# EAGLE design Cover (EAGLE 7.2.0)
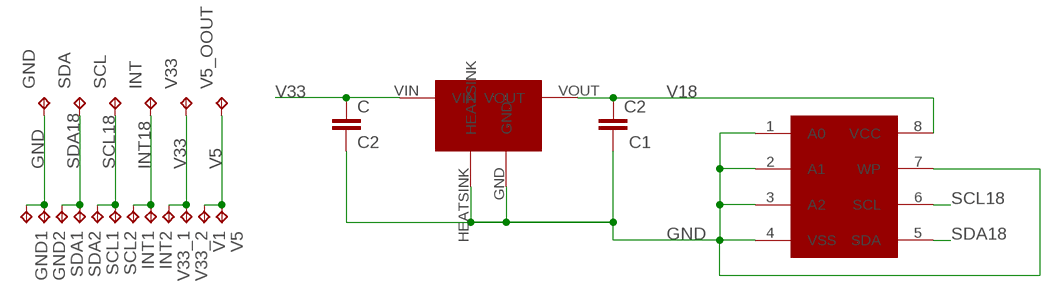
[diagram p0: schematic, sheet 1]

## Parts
C  C2  C-EUC0603  [C0603]
C2  C1  C-EUC0603  [C0603]
GND  TPTP20SQ  [TP20SQ]
GND1  TPTP20SQ  [TP20SQ]
GND2  TPTP20SQ  [TP20SQ]
INT  TPTP20SQ  [TP20SQ]
INT1  TPTP20SQ  [TP20SQ]
INT2  TPTP20SQ  [TP20SQ]
SCL  TPTP20SQ  [TP20SQ]
SCL1  TPTP20SQ  [TP20SQ]
SCL2  TPTP20SQ  [TP20SQ]
SDA  TPTP20SQ  [TP20SQ]
SDA1  SDA  TPTP20SQ  [TP20SQ]
SDA2  SDA  TPTP20SQ  [TP20SQ]
U$1  CAT24  [CAT24]
U$2  MCP1700-DFN6  [DFN6-2X2]
V1  V5  TPTP20SQ  [TP20SQ]
V5  V5  TPTP20SQ  [TP20SQ]
V5_OOUT  TPTP20SQ  [TP20SQ]
V33  TPTP20SQ  [TP20SQ]
V33_1  TPTP20SQ  [TP20SQ]
V33_2  TPTP20SQ  [TP20SQ]

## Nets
GND: C2.2 C.2 GND1.TP GND2.TP GND.TP U$1.1(A0) U$1.2(A1) U$1.3(A2) U$1.4(VSS) U$1.7(WP) U$2.GND U$2.HEATSINK
INT18: INT1.TP INT2.TP INT.TP
SCL18: SCL1.TP SCL2.TP SCL.TP U$1.6(SCL)
SDA18: SDA1.TP SDA2.TP SDA.TP U$1.5(SDA)
V5: V1.TP V5.TP V5_OOUT.TP
V18: C2.1 U$1.8(VCC) U$2.VOUT
V33: C.1 U$2.VIN V33.TP V33_1.TP V33_2.TP

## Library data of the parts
C C2 = rcl:C-EU: CAPACITOR, European symbol
GND GND1 GND2 INT INT1 INT2 SCL SCL1 SCL2 SDA SDA1 SDA2 V1 V5 V5_OOUT V33 V33_1 V33_2 = testpad:TP: Test pad
U$1 = cat24:CAT24
U$2 = MCP1700_DFN6-2x2:MCP1700-DFN6

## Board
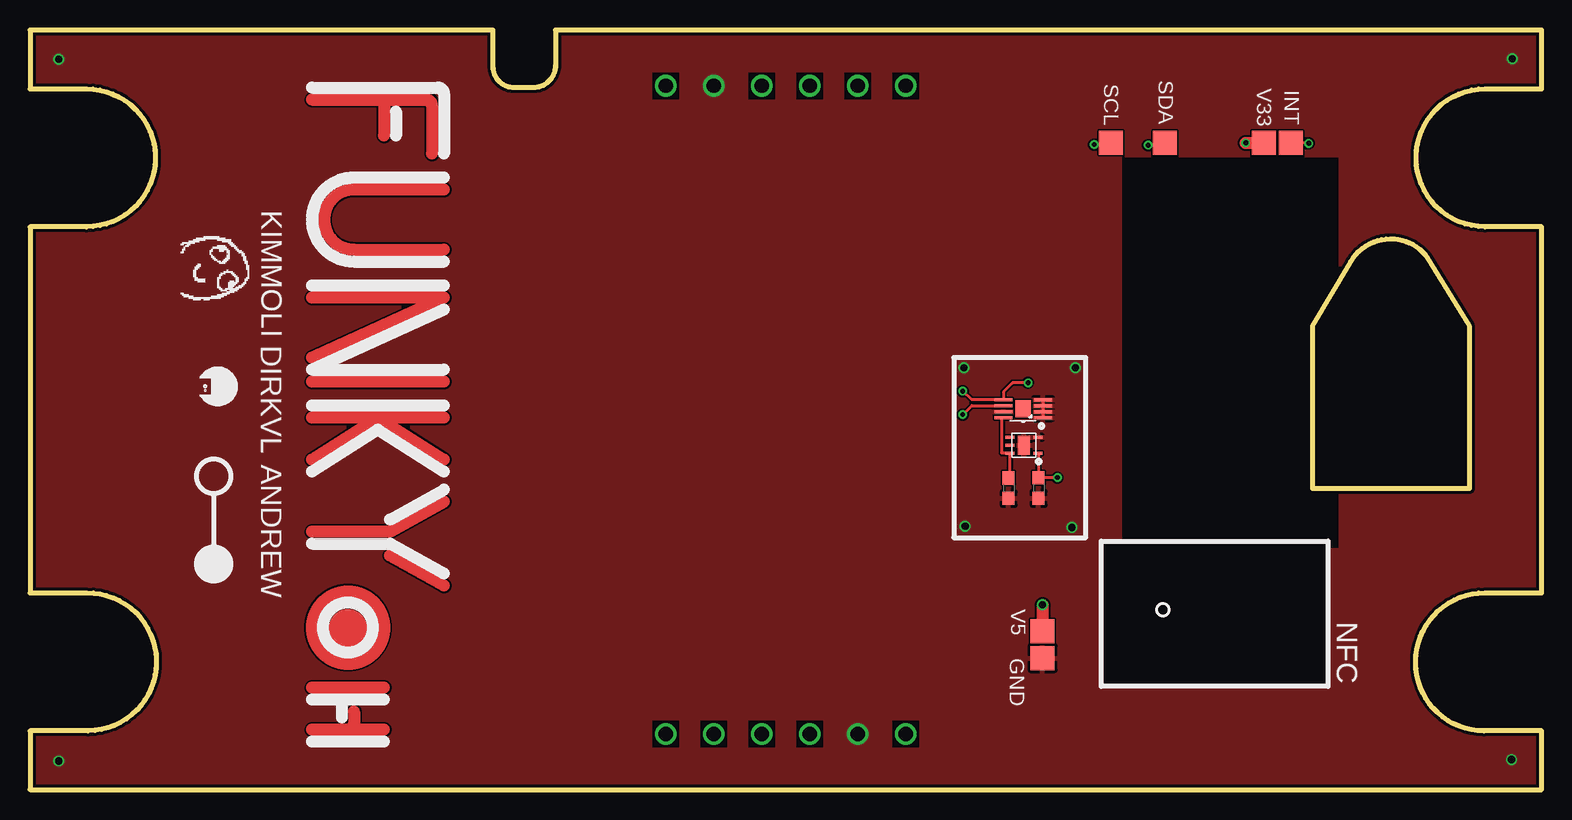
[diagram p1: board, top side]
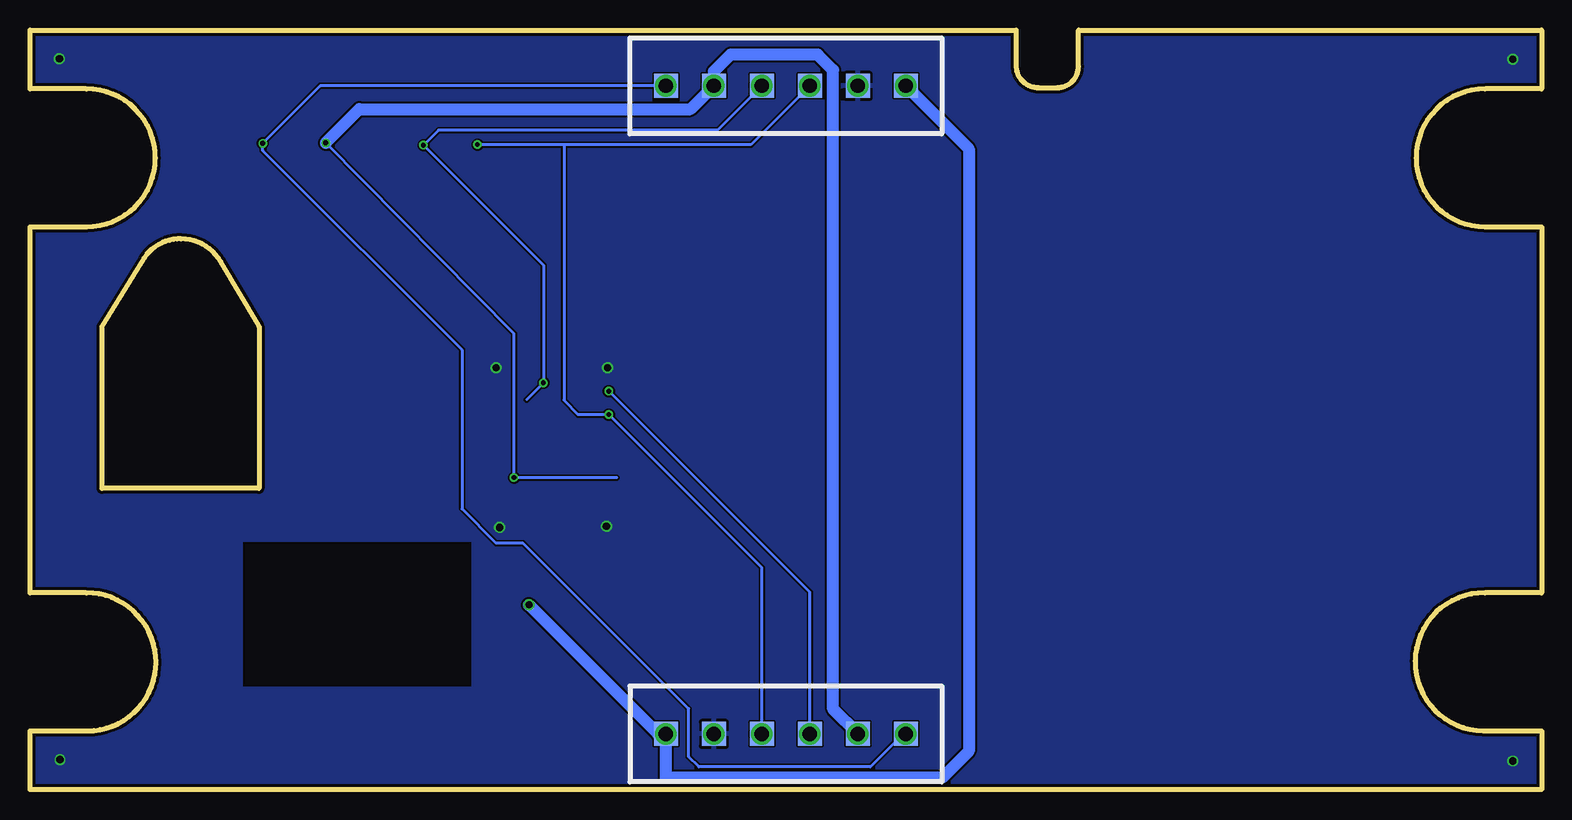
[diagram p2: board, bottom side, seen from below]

Size 126 x 63.3 mm. Coordinates in mm from the lower left corner, seen from the top.
Outline: 0,0 126,0 126,4.9 121.2,4.9 arc-90 115.5,10.6 arc-90 121.3,16.4 126,16.4 126,46.9 121.3,46.9 arc-180 121.3,58.4 126,58.4 126,63.3 43.8,63.3 43.8,60.35 arc-90 41.95,58.5 40.35,58.5 arc-90 38.6,60.25 38.6,63.3 0,63.3 0,58.4 4.7,58.4 arc-180 4.7,46.9 0,46.9 0,16.4 4.72,16.4 arc-180 4.85,4.9 0,4.9 0,0
Outline: 106.9,38.6 106.9,25.1 120,25.1 120,38.6 116.5,44.3 arc56 113.4,45.9 arc59 110.1,44 106.9,38.6
Copper layers (1*16): Top 0.035mm / dielectric 1.5mm / Bottom 0.035mm
Design rules "ITEADstudio_DRC": minimum track width 6mil, minimum drill 12mil, track to track 6mil, track to pad 6mil, pad to pad 6mil, via to via 6mil, smd to smd 0mil, copper to edge 10mil, drill to drill 10mil, minimum pad ring 10mil, minimum via ring 6mil, stop-mask expansion 2mil, vias tented up to drill 100mil, thermal gap 10mil
tRestrict: area 51.9,3.6 to 54.1,5.8; area 55.9,3.6 to 58.1,5.8; area 59.9,3.6 to 62.1,5.8; area 63.9,3.6 to 66.1,5.8; area 71.9,3.6 to 74.1,5.8; area 51.9,57.5 to 54.1,59.8; area 59.9,57.5 to 62.1,59.8; area 63.9,57.5 to 66.1,59.8; area 67.9,57.5 to 70.1,59.8; area 71.9,57.5 to 74.1,59.8; area 89.2,8.6 to 108.2,20.6; area 91,20.1 to 109,52.6
bRestrict: area 89.2,8.6 to 108.2,20.6

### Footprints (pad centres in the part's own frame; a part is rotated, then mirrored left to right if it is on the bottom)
C0603 = smd 1.1 x 1: 1 -0.85,0; 2 0.85,0
TP20SQ = smd 2 x 2: TP 0,0
CAT24 = smd 0.25 x 1.5: 1 -0.75,-1.65; 2 -0.25,-1.65; 3 0.25,-1.65; 4 0.75,-1.65; 5 0.75,1.65; 6 0.25,1.65; 7 -0.25,1.65; 8 -0.75,1.65 | smd 1.4 x 1.3: P$1 0,0
DFN6-2X2 = smd 0.75 x 0.25: GND -1.15,-0.65; P$1 1.15,0; P$2 1.15,-0.65; VIN -1.15,0.65; VOUT 1.15,0.65 | smd 1 x 1.6: HEATSINK 0,0

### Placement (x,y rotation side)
C  84.08,25.13 270 top
C2  81.58,25.12 270 top
GND  84.4,10.95 0 top
GND1  57,58.65 0 bottom
GND2  69,4.65 0 bottom
INT  105.1,53.9 180 top
INT1  73,58.65 0 bottom
INT2  53,4.65 0 bottom
SCL  90.1,53.9 180 top
SCL1  61,58.65 0 bottom
SCL2  65,4.65 0 bottom
SDA  94.6,53.9 180 top
SDA1  65,58.65 0 bottom
SDA2  61,4.65 0 bottom
U$1  82.8,31.75 90 top
U$2  82.85,28.7 180 top
U$3  [FUNKY]  23.5,32.5 270 top
U$4  DAFUG  [DAFUG]  15.18,43.25 270 top
V1  53,58.65 0 bottom
V5  84.4,13.2 0 top
V5_OOUT  73,4.65 0 bottom
V33  102.85,53.9 180 top
V33_1  69,58.65 0 bottom
V33_2  57,4.65 0 bottom

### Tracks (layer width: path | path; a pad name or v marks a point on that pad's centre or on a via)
GND  (via drill 0.6, 1.2)
  Top 0.254: U$1.4 U$1.3 U$1.2 U$1.1
  other vias: 69,4.65 57,58.65 2.4,60.85 2.4,2.38 123.5,2.5 123.55,60.9 77.85,35.15 87.15,35.15 77.95,21.95 86.85,21.85
  pour Bottom: 0,0 126,0 126,63.3 0,63.3
  pour Top: 0,0 126,0 126,63.3 0,63.3
INT18  (via drill 0.4, 1.2)
  Top 0.254: v106.6,53.85 INT.TP
  Bottom 0.254: INT1.TP 101.8,58.65 v106.6,53.85 106.6,53.25 90,36.65 90,23.4 87.15,20.55 84.9,20.55 71.1,6.75 71.1,2.75 70.25,1.9 55.95,1.9 52.9,4.95
  Bottom 0.406: 52.9,4.95 INT2.TP
  other vias: 53,4.65 73,58.65
SCL18  (via drill 0.4, 1.2)
  Top 0.254: v77.75,31.25 78.5,32 U$1.6 | v88.7,53.75 89.5,53.8 SCL.TP
  Bottom 0.254: 81.5,53.75 81.5,32.45 80.3,31.25 v77.75,31.25 65,18.5 SCL2.TP | SCL1.TP 65.9,53.75 81.5,53.75 | 81.5,53.75 v88.7,53.75
  other vias: 65,4.65 61,58.65
SDA18  (via drill 0.4, 1.2)
  Top 0.254: v77.75,33.2 78.5,32.5 U$1.5 81.15,33.15 81.9,33.9 v83.2,33.9 | v93.2,53.7 SDA.TP
  Bottom 0.254: 84.6,32.5 v83.2,33.9 83.2,43.7 v93.2,53.7 91.95,54.95 68.7,54.95 SDA1.TP | SDA2.TP 61,16.45 v77.75,33.2
  other vias: 61,4.65 65,58.65
V5  (via drill 0.6, 1.2)
  Top 1.016: v84.4,15.4 V5.TP
  Bottom 1.016: V1.TP 47.75,53.4 47.75,3.2 49.95,1 73,1 V5_OOUT.TP 73.65,4.65 v84.4,15.4
  other vias: 73,4.65 53,58.65
V18
  Top 0.254: C2.1 81.7,25.57 U$2.VOUT 81,28.05 81,31 U$1.8
V33  (via drill 0.4, 1.2)
  Top 0.254: U$2.VIN 84.08,28.05 C.1 84.1,26 v85.65,26
  Top 1.016: v101.35,53.9 V33.TP
  Bottom 0.254: 77.1,26 v85.65,26 85.65,38 v101.35,53.9
  Bottom 1.016: v101.35,53.9 98.55,56.7 70.95,56.7 V33_1.TP 69,59.85 67.6,61.25 60.35,61.25 59.05,59.95 59.05,6.7 V33_2.TP
  other vias: 57,4.65 69,58.65
(copper drawn outside any net)
  shapes: Top circle x1

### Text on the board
tPlace: KIMMOLI | DIRKVL | ANDREW | NFC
